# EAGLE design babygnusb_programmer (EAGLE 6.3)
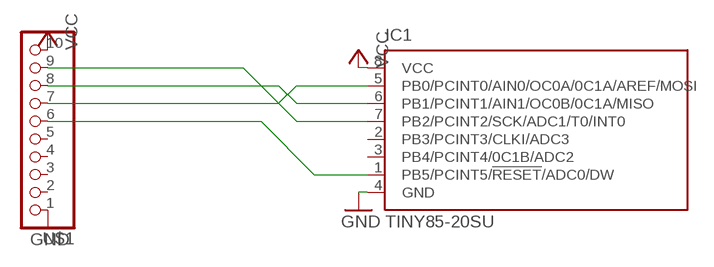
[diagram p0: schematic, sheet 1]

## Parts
IC1  TINY85-20SU  [8S2]
U$1  10-PIN-SMD-2.54  [10PIN-SMD-2.54]

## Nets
GND: IC1.4(GND) U$1.1
N$1: IC1.7(PB2/PCINT2/SCK/ADC1/T0/INT0) U$1.9
N$2: IC1.6(PB1/PCINT1/AIN1/OC0B/0C1A/MISO) U$1.8
N$3: IC1.5(PB0/PCINT0/AIN0/OC0A/0C1A/AREF/MOSI) U$1.7
N$4: IC1.1(PB5/PCINT5/!RESET!/ADC0/DW) U$1.6
VCC: IC1.8(VCC) U$1.10
Unconnected: IC1.2(PB3/PCINT3/CLKI/ADC3) IC1.3(PB4/PCINT4/0C1B/ADC2) U$1.2 U$1.3 U$1.4 U$1.5

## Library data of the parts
IC1 = anyma-lib:TINY85: 8-bit AVR Microcontroller with 1K Bytes In-System Programmable Flash Source: http://www.atmel.com/dyn/resources/prod_documents/2535S.pdf; MPN: ATTINY13-20SU; OC_FARNELL: 9171568; OC_NEWARK: 96K6522
U$1 = anyma-lib:10-PIN-SMD-2.54

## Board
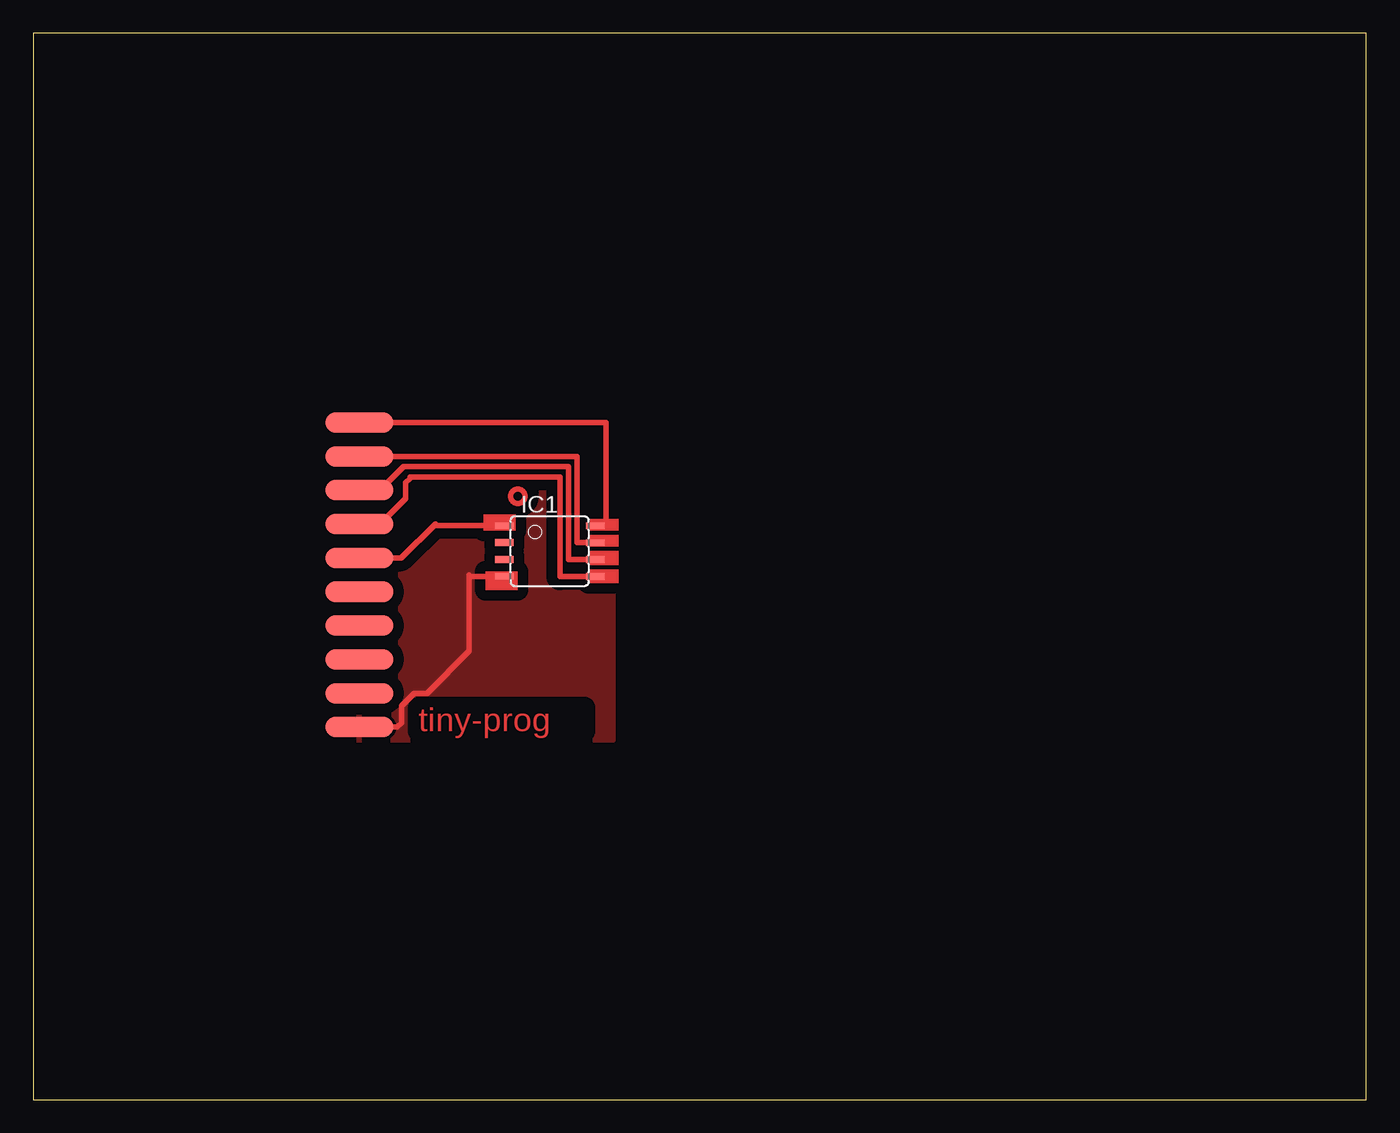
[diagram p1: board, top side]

Size 100 x 80 mm. Coordinates in mm from the lower left corner, seen from the top.
Outline: 0,0 100,0 100,80 0,80 0,0
Copper layers (1*16): Top 0.035mm / dielectric 1.5mm / Bottom 0.035mm
Design rules "default": minimum track width 10mil, minimum drill 24mil, track to track 8mil, track to pad 8mil, pad to pad 8mil, via to via 8mil, smd to smd 8mil, copper to edge 40mil, drill to drill 8mil, minimum pad ring 10mil, minimum via ring 8mil, stop-mask expansion 4mil, vias tented up to drill 0mil, thermal gap 10mil

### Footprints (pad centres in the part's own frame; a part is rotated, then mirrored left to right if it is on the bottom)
8S2 = smd 0.5 x 1.4: 1 -1.905,-3.404; 2 -0.645,-3.404; 3 0.625,-3.404; 4 1.895,-3.404; 5 1.905,3.404; 6 0.635,3.404; 7 -0.635,3.404; 8 -1.905,3.404
10PIN-SMD-2.54 = smd 5.08 x 1.524: 1 0,8.89; 2 0,6.35; 3 0,3.81; 4 0,1.27; 5 0,-1.27; 6 0,-3.81; 7 0,-6.35; 8 0,-8.89; 9 0,-11.43; 10 0,-13.97

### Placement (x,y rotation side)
IC1  38.75,41.15 270 top
U$1  24.45,36.83 180 top

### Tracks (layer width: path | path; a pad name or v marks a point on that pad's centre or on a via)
GND
  Top 0.406: U$1.1 27.3,27.94 27.62,28.26 27.62,29.53 28.57,30.48 29.53,30.48 32.7,33.66 32.7,39.25 | 32.7,39.37 32.7,39.26 32.7,39.25 | IC1.4 32.7,39.25
  pour Top (isolate 0.813): 23.5,51.75 43.5,51.75 43.5,26.99 23.5,26.99
N$1
  Top 0.406: U$1.9 40.79,48.26 40.79,41.78 IC1.7
N$2
  Top 0.406: U$1.8 24.85,46.12 26.4,46.12 27.77,47.49 40.12,47.49 40.15,47.46 40.15,40.8 40.15,40.64 40.15,40.51 IC1.6
N$3
  Top 0.406: U$1.7 24.94,42.69 25.55,42.69 27.95,45.09 27.95,46.29 28.26,46.6 28.26,46.7 39.52,46.7 39.52,39.24 IC1.5
N$4
  Top 0.406: U$1.6 27.59,40.64 30.16,43.18 30.16,43.05 IC1.1
VCC
  Top 0.406: U$1.10 42.98,50.8 42.98,43.05 IC1.8
(copper drawn outside any net)
  shapes: Top area x6, Top circle x1

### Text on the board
Top: tiny-prog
